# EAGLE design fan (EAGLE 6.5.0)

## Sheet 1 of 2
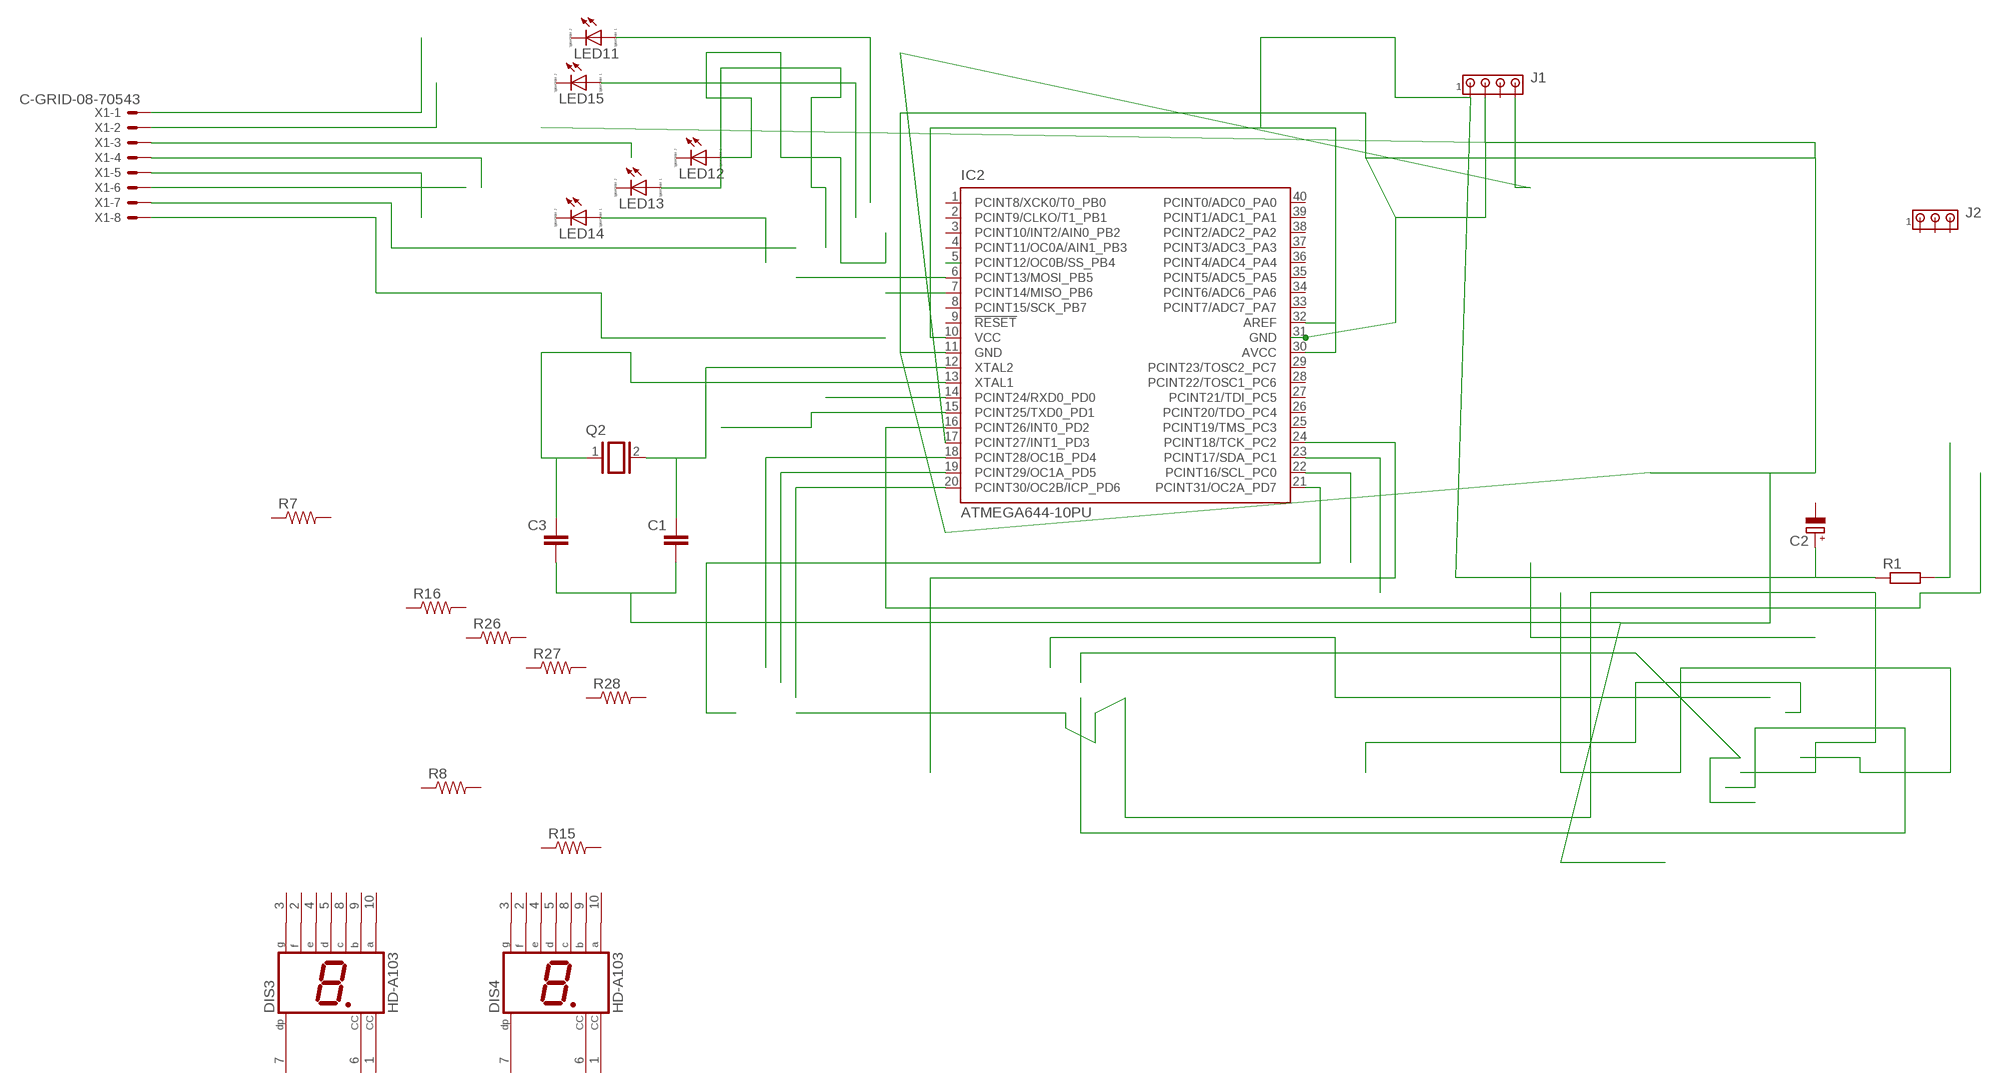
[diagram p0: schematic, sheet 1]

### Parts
C1  C-EU025-030X050  [C025-030X050]
C2  CPOL-EUE2,5-6E  [E2,5-6E]
C3  C-EU025-030X050  [C025-030X050]
DIS3  HD-A103  [HDSP-A]
DIS4  HD-A103  [HDSP-A]
IC2  ATMEGA644-10PU  [DIL40]
J1  MTA04-100  [10X04MTA]
J2  MTA03-100  [10X03MTA]
LED11  LED_ELD260  [LED_LD260]
LED12  LED_ELD260  [LED_LD260]
LED13  LED_ELD260  [LED_LD260]
LED14  LED_ELD260  [LED_LD260]
LED15  LED_ELD260  [LED_LD260]
Q2  XTAL/S  [QS]
R1  R-EU_0204/7  [0204/7]
R7  R-US_0204/7  [0204/7]
R8  R-US_0204/7  [0204/7]
R15  R-US_0204/7  [0204/7]
R16  R-US_0204/7  [0204/7]
R26  R-US_0204/7  [0204/7]
R27  R-US_0204/7  [0204/7]
R28  R-US_0204/7  [0204/7]
X1  C-GRID-08-70543  [70543-08]

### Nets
N$1: R1.2
N$2: C3.1 IC2.13(XTAL1) Q2.1
N$3: IC2.16(PCINT26/INT0_PD2)
N$4: C1.1 IC2.12(XTAL2) Q2.2
N$5: LED15.A
N$6: IC2.6(PCINT13/MOSI_PB5)
N$7: C2.+ IC2.10(VCC) IC2.30(AVCC) IC2.32(AREF) J1.1 R1.1
N$8: IC2.7(PCINT14/MISO_PB6)
N$9: LED14.A
N$11: X1.1
N$12: LED13.A
N$13: LED12.A
N$14: IC2.18(PCINT28/OC1B_PD4)
N$15: IC2.19(PCINT29/OC1A_PD5)
N$16: IC2.20(PCINT30/OC2B/ICP_PD6)
N$18: IC2.15(PCINT25/TXD0_PD1)
N$22: X1.2
N$24: X1.8
N$28: IC2.23(PCINT17/SDA_PC1)
N$30: LED11.A
N$31: IC2.14(PCINT24/RXD0_PD0)
N$36: X1.4
N$37: X1.5
N$38: X1.7
N$39: X1.3
N$40: X1.6
N$42: IC2.17(PCINT27/INT1_PD3) J1.4
N$43: C1.2 C3.2 IC2.11(GND) IC2.31(GND) J1.2
N$45: IC2.24(PCINT18/TCK_PC2)
N$46: IC2.22(PCINT16/SCL_PC0)
N$53: IC2.21(PCINT31/OC2A_PD7)
N$56: IC2.5(PCINT12/OC0B/SS_PB4)
Unconnected: C2.- DIS3.1(CC) DIS3.2(F) DIS3.3(G) DIS3.4(E) DIS3.5(D) DIS3.6(CC) DIS3.7(DP) DIS3.8(C) DIS3.9(B) DIS3.10(A) DIS4.1(CC) DIS4.2(F) DIS4.3(G) DIS4.4(E) DIS4.5(D) DIS4.6(CC) DIS4.7(DP) DIS4.8(C) DIS4.9(B) DIS4.10(A) IC2.1(PCINT8/XCK0/T0_PB0) IC2.2(PCINT9/CLKO/T1_PB1) IC2.3(PCINT10/INT2/AIN0_PB2) IC2.4(PCINT11/OC0A/AIN1_PB3) IC2.8(PCINT15/SCK_PB7) IC2.9(!RESET) IC2.25(PCINT19/TMS_PC3) IC2.26(PCINT20/TDO_PC4) IC2.27(PCINT21/TDI_PC5) IC2.28(PCINT22/TOSC1_PC6) IC2.29(PCINT23/TOSC2_PC7) IC2.33(PCINT7/ADC7_PA7) IC2.34(PCINT6/ADC6_PA6) IC2.35(PCINT5/ADC5_PA5) IC2.36(PCINT4/ADC4_PA4) IC2.37(PCINT3/ADC3_PA3) IC2.38(PCINT2/ADC2_PA2) IC2.39(PCINT1/ADC1_PA1) IC2.40(PCINT0/ADC0_PA0) J1.3 J2.1 J2.2 J2.3 LED11.K(C) LED12.K(C) LED13.K(C) LED14.K(C) LED15.K(C) R7.1 R7.2 R8.1 R8.2 R15.1 R15.2 R16.1 R16.2 R26.1 R26.2 R27.1 R27.2 R28.1 R28.2

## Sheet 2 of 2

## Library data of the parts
C1 C3 = resistor:C-EU: CAPACITOR, European symbol
C2 = rcl:CPOL-EU: POLARIZED CAPACITOR, European symbol
DIS3 DIS4 = display-hp:HD-A103: LED DISPLAY 1-character 7 segment, decimal point right; OC_FARNELL: unknown; OC_NEWARK: unknown
IC2 = atmel:ATMEGA644-*PU: 8-bit Microcontroller with 64K Bytes In-System Programmable Flash Auto generated by make-symbol-device-package-bsdl.ulp Rev. 34 Source: http://www.atmel.com/dyn/resources/prod_documents/doc2593.pdf; MPN: ATMEGA644V-10PU; OC_FARNELL: 1288342; OC_NEWARK: 23M5062
J1 = con-amp:MTA04-100: AMP connector
J2 = con-amp:MTA03-100: AMP connector
LED11-LED15 = eagle-ltspice:LED_E: LED; SPICEMODEL: NONE; SPICEPREFIX: D; SPICETYPE: diode
Q2 = special:XTAL/S: CRYSTAL
R1 = rcl:R-EU_: RESISTOR, European symbol
R7 R8 R15 R16 R26-R28 = rcl:R-US_: RESISTOR, American symbol
X1 = con-molex:C-GRID-08: CONNECTOR wire to board 2.54 mm (0.100") pitch header; OC_FARNELL: unknown; OC_NEWARK: unknown

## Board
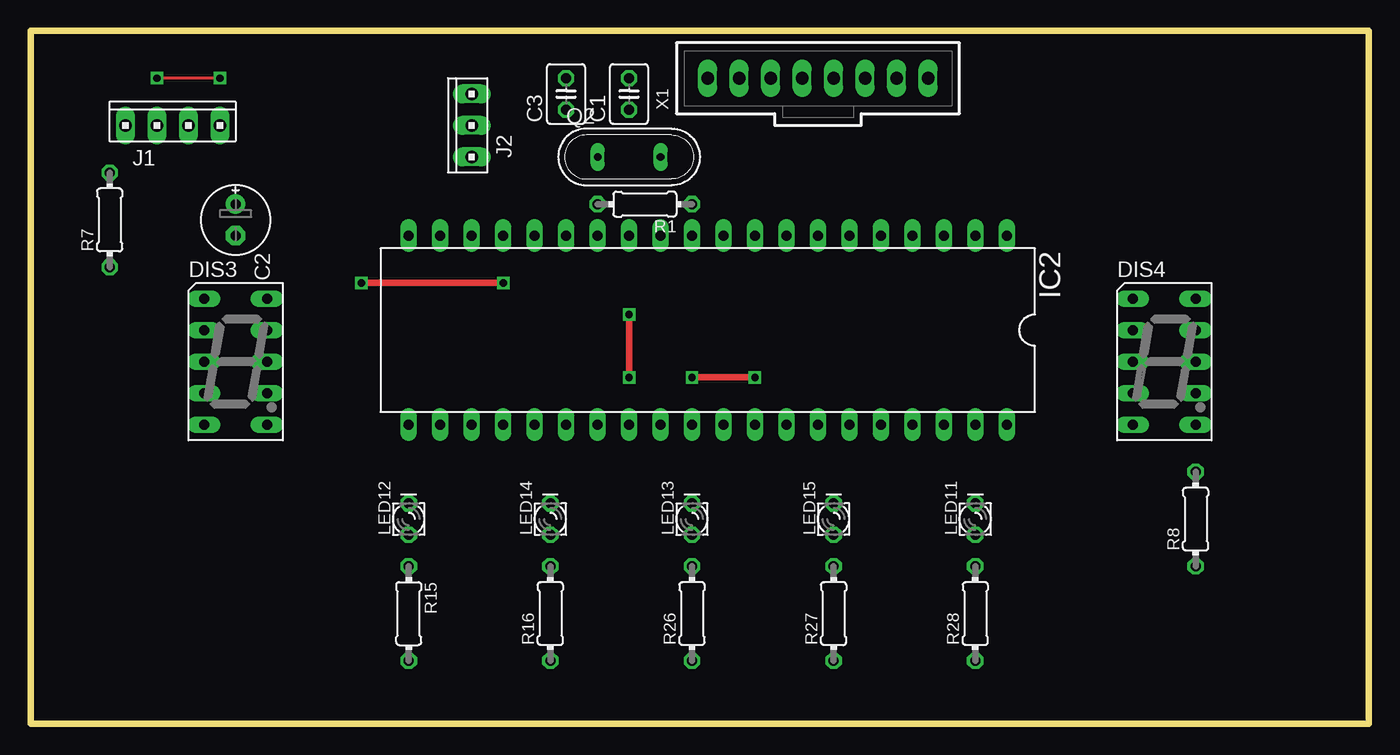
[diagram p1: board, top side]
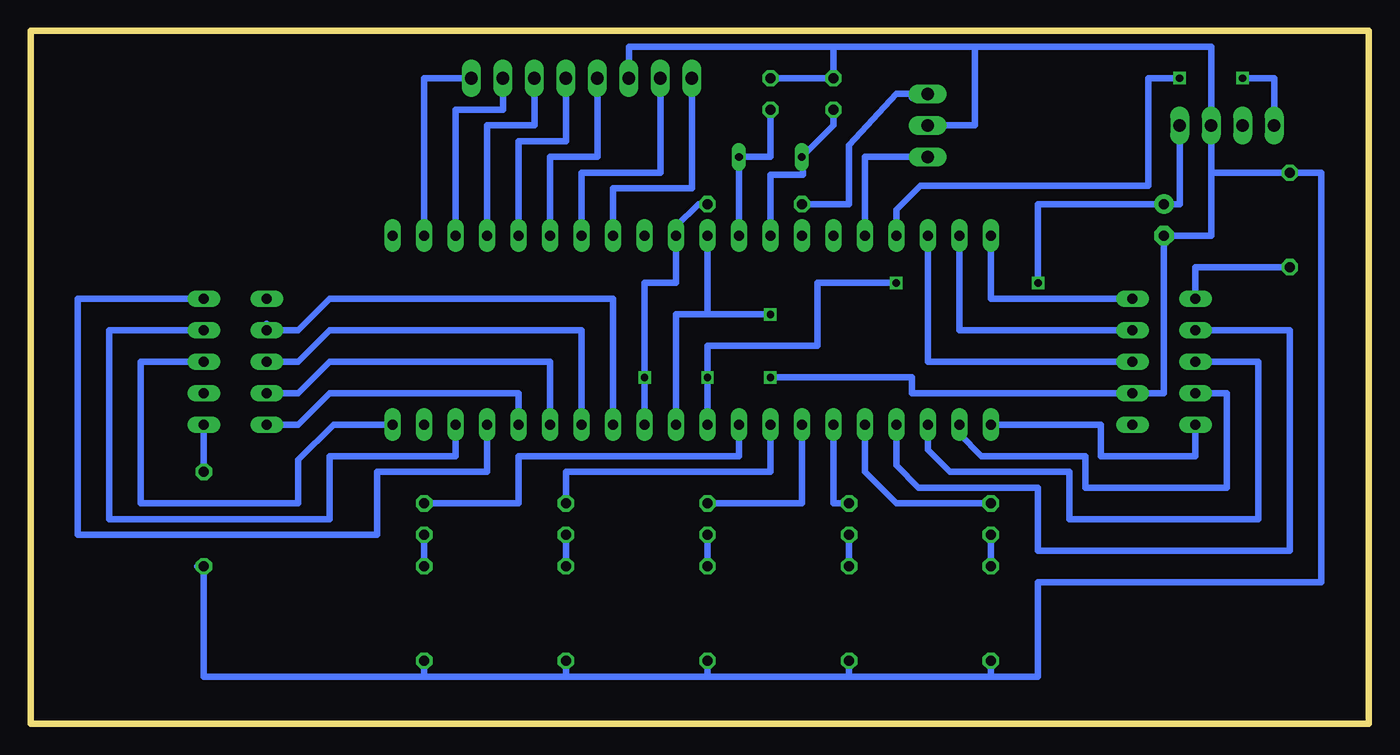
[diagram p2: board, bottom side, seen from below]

Size 107.93 x 55.88 mm. Coordinates in mm from the lower left corner, seen from the top.
Outline: 107.93,0 107.93,55.88 0,55.88 0,0 107.93,0
Copper layers (1*16): Top 0.035mm / dielectric 1.5mm / Bottom 0.035mm
Design rules "default": minimum track width 10mil, minimum drill 24mil, track to track 8mil, track to pad 8mil, pad to pad 8mil, via to via 8mil, smd to smd 8mil, copper to edge 40mil, drill to drill 8mil, minimum pad ring 10mil, minimum via ring 8mil, stop-mask expansion 4mil, vias tented up to drill 0mil, thermal gap 10mil

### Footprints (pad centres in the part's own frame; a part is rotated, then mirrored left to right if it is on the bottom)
C025-030X050 = drill 0.813 octagon: 1 -1.27,0; 2 1.27,0
E2,5-6E = drill 0.813 pad 1.575: + -1.27,0 | drill 0.813 pad 1.575 octagon: - 1.27,0
HDSP-A = drill 0.813 long: 1 -2.54,5.08; 2 -2.54,2.54; 3 -2.54,0; 4 -2.54,-2.54; 5 -2.54,-5.08; 6 2.54,-5.08; 7 2.54,-2.54; 8 2.54,0; 9 2.54,2.54; 10 2.54,5.08
DIL40 = drill 0.813 long: 1 -24.13,-7.62; 2 -21.59,-7.62; 3 -19.05,-7.62; 4 -16.51,-7.62; 5 -13.97,-7.62; 6 -11.43,-7.62; 7 -8.89,-7.62; 8 -6.35,-7.62; 9 -3.81,-7.62; 10 -1.27,-7.62; 11 1.27,-7.62; 12 3.81,-7.62; 13 6.35,-7.62; 14 8.89,-7.62; 15 11.43,-7.62; 16 13.97,-7.62; 17 16.51,-7.62; 18 19.05,-7.62; 19 21.59,-7.62; 20 24.13,-7.62; 21 24.13,7.62; 22 21.59,7.62; 23 19.05,7.62; 24 16.51,7.62; 25 13.97,7.62; 26 11.43,7.62; 27 8.89,7.62; 28 6.35,7.62; 29 3.81,7.62; 30 1.27,7.62; 31 -1.27,7.62; 32 -3.81,7.62; 33 -6.35,7.62; 34 -8.89,7.62; 35 -11.43,7.62; 36 -13.97,7.62; 37 -16.51,7.62; 38 -19.05,7.62; 39 -21.59,7.62; 40 -24.13,7.62
10X04MTA = drill 1.016 long: 1 3.81,0; 2 1.27,0; 3 -1.27,0; 4 -3.81,0
10X03MTA = drill 1.016 long: 1 2.54,0; 2 0,0; 3 -2.54,0
LED_LD260 = drill 0.813 octagon: A -1.27,0; K 1.27,0
QS = drill 0.61 long: 1 -2.54,0; 2 2.54,0
0204/7 = drill 0.813 octagon: 1 -3.81,0; 2 3.81,0
70543-08 = drill 1.016 long: 1 -8.89,0; 2 -6.35,0; 3 -3.81,0; 4 -1.27,0; 5 1.27,0; 6 3.81,0; 7 6.35,0; 8 8.89,0

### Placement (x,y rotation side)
C1  48.26,50.8 90 top
C2  16.51,40.64 270 top
C3  43.18,50.8 90 top
DIS3  16.51,29.21 0 top
DIS4  91.44,29.21 0 top
IC2  54.61,31.75 180 top
J1  11.43,48.26 0 top
J2  35.56,48.26 90 top
LED11  76.2,16.51 90 top
LED12  30.48,16.51 90 top
LED13  53.34,16.51 90 top
LED14  41.91,16.51 90 top
LED15  64.77,16.51 90 top
Q2  48.26,45.72 0 top
R1  49.53,41.91 180 top
R7  6.35,40.64 90 top
R8  93.98,16.51 90 top
R15  30.48,8.89 270 top
R16  41.91,8.89 90 top
R26  53.34,8.89 90 top
R27  64.77,8.89 90 top
R28  76.2,8.89 90 top
X1  63.5,52.07 0 top

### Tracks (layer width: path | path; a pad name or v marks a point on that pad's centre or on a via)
N$1
  Bottom 0.508: 35.56,50.8 38.1,50.8 41.91,46.65 41.91,41.91 R1.2 | 35.56,50.8 35.56,50.5 36.83,50.5 35.56,50.8
N$2
  Bottom 0: 45.64,44.26 48.26,44.45 48.26,44.26 48.26,43.71 48.26,43.18
  Bottom 0.508: C3.1 43.18,48.26 Q2.1 45.64,44.26 48.26,44.26 48.26,43.71 IC2.13
N$3
  Bottom 0.508: 35.26,45.72 40.64,45.72 IC2.16
N$4
  Bottom 0.508: C1.1 48.26,45.72 Q2.2 IC2.12
N$7  (via drill 0.6)
  Top 0.508: v38.1,35.56 v26.67,35.56 | v53.34,27.94 v58.42,27.94
  Bottom 0.508: R1.1 54.08,41.91 55.88,40.11 IC2.10 55.88,35.56 58.42,35.56 v58.42,27.94 IC2.32 | J1.1 15.24,41.91 C2.+ 26.67,41.91 v26.67,35.56 | v38.1,35.56 44.45,35.56 44.45,30.48 53.34,30.48 v53.34,27.94 IC2.30
N$10
  Bottom 0.508: 43.18,24.13 43.18,17.78 41.91,17.78 | 45.72,24.13 45.72,17.78 53.34,17.78 | 50.8,24.13 50.8,21.59 68.58,21.59 68.58,17.78 76.2,17.78 | 48.26,24.13 48.26,20.32 64.77,20.32 64.77,17.78 | 40.64,24.13 40.64,20.32 38.1,17.78 30.48,17.78
N$14
  Bottom 0.508: 35.56,37.89 IC2.18 35.56,29.21 19.05,29.21
N$15
  Bottom 0.508: IC2.19 33.02,31.75 19.05,31.75
N$17
  Bottom 0.508: 93.98,24.13 93.98,20.32
N$19
  Bottom 0.508: 13.97,34.29 13.97,36.83 6.35,36.83
N$20
  Bottom 0.508: 13.97,29.21 8.89,29.21 8.89,16.51 24.13,16.51
N$21
  Bottom 0.508: 21.59,21.59 13.97,21.59 13.97,24.13
N$23
  Bottom 0.508: 41.91,15.24 41.91,12.7 | 53.34,15.24 53.34,12.7 | 64.77,15.24 64.77,12.7 | 76.2,15.24 76.2,12.7 | 30.48,15.24 30.48,12.7
N$25
  Bottom 0.508: 10.16,44.45 12.7,44.45
N$26
  Bottom 0.508: 88.9,31.75 86.36,31.75 83.82,34.29 60.96,34.29 60.96,24.13
N$27
  Bottom 0.508: 35.56,48.26 31.75,48.26 31.75,54.61
N$28
  Bottom 0.508: IC2.23 35.56,22.12 33.76,20.32 24.13,20.32 24.13,16.51
N$29
  Bottom 0.508: 88.9,29.21 86.36,29.21 83.82,31.75 63.5,31.75 63.5,24.13
N$33
  Bottom 0.508: 83.82,26.67 68.58,26.67 68.58,24.13
N$34
  Bottom 0.508: 88.9,26.67 86.36,26.67 83.82,29.21 66.04,29.21 66.04,24.13
N$35
  Bottom 0.508: 71.12,24.13 71.12,20.32 80.01,20.32 80.01,15.24 90.17,15.24
N$41
  Bottom 0.508: 88.9,31.75 89.64,31.75 88.9,32.28 88.9,31.75
N$42  (via drill 0.6)
  Top 0.254: v15.24,52.07 v10.16,52.07
  Bottom 0.508: IC2.17 38.1,41.44 36.14,43.4 17.78,43.4 17.78,45.72 17.78,52.07 v15.24,52.07 | v10.16,52.07 7.62,52.07 J1.4
N$43  (via drill 0.6)
  Top 0.508: v48.26,33.02 v48.26,27.94
  Bottom 0.508: C1.2 C3.2 43.18,54.61 | 59.69,52.07 59.69,54.61 43.18,54.61 | 43.18,54.61 12.7,54.61 J1.2 12.7,39.37 16.51,39.37 16.51,26.67 36.83,26.67 36.83,27.94 v48.26,27.94 | 53.34,33.02 55.88,33.02 IC2.31 | IC2.11 53.34,33.02 | 53.34,33.02 v48.26,33.02
N$44
  Bottom 0.508: 73.66,24.13 73.66,21.59 83.82,21.59 83.82,16.51 97.79,16.51
N$45
  Bottom 0.508: 38.47,24.5 IC2.24 38.1,20.85 36.3,19.05 26.67,19.05 26.67,13.97
N$46
  Bottom 0.508: IC2.22 33.02,23.39 31.22,21.59 22.86,21.59 22.86,19.05
N$47
  Bottom 0.508: 78.74,24.13 83.52,24.13 86.36,21.29 86.36,17.78 90.17,17.78
N$48
  Bottom 0.508: 90.17,17.78 99.06,17.78 99.06,29.21 93.98,29.21
N$49
  Bottom 0.508: 93.98,31.75 101.6,31.75 101.6,16.51 97.79,16.51
N$50
  Bottom 0.508: 90.17,15.24 104.14,15.24 104.14,34.29 93.98,34.29
N$51
  Bottom 0.508: 83.82,26.67 86.36,24.13 88.9,24.13 | 76.2,3.81 76.2,5.08 | 30.48,3.81 30.48,5.08 | 53.34,3.81 53.34,5.08 | 64.77,3.81 64.77,5.08 | 41.91,3.81 41.91,5.08
N$52
  Bottom 0.508: 13.97,26.67 11.43,26.67 11.43,19.05 22.86,19.05
N$53
  Bottom 0.508: IC2.21 21.59,24.13 21.59,21.59
N$54
  Bottom 0.508: 13.97,31.75 6.35,31.75 6.35,13.97 26.67,13.97
N$55
  Bottom 0.508: 10.16,44.45 3.81,44.45 3.81,11.43 26.67,11.43 26.67,3.81 93.98,3.81 93.98,12.7 94.51,12.7
N$57
  Bottom 0.508: 88.9,26.67 88.6,26.67 88.9,26.97 88.9,26.67
N$58
  Bottom 0.508: 54.61,52.07 54.61,43.18 60.96,43.18 60.96,39.37
N$59
  Bottom 0.508: 72.39,52.07 76.2,52.07 76.2,39.37
N$60
  Bottom 0.508: 69.85,52.07 69.85,49.53 73.66,49.53 73.66,39.37
N$61
  Bottom 0.508: 67.31,52.07 67.31,48.26 71.12,48.26 71.12,39.37
N$62
  Bottom 0.508: 64.77,52.07 64.77,46.99 68.58,46.99 68.58,39.37
N$63
  Bottom 0.508: 62.23,52.07 62.23,45.72 66.04,45.72 66.04,39.37
N$64
  Bottom 0.508: 63.5,39.37 63.5,44.45 57.15,44.45 57.15,52.07
N$65
  Bottom 0.508: 19.05,34.29 30.48,34.29 30.48,39.37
